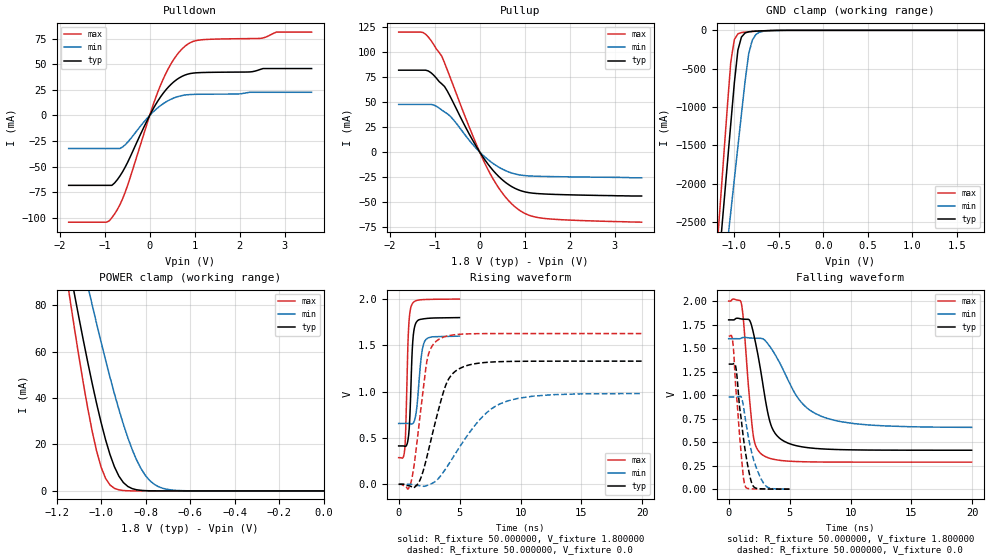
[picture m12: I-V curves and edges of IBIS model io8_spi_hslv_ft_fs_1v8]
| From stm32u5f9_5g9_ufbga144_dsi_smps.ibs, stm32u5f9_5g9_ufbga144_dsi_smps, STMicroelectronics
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|   Model io8_spi_hslv_ft_fs_1v8
[Model]  io8_spi_hslv_ft_fs_1v8
Model_type I/O
Polarity   Non-Inverting
Enable   Active-Low
Vinl =   0.540000V
Vinh =   1.260000V
Vmeas =  0.900000V
Cref =   50.000000pF
Rref =   100.000000M
Vref =   0.0V
C_comp   3.338700pF   3.332500pF   3.379000pF
[Temperature Range]   25.000000   0.140000k   -40.000000
[Pullup Reference]   1.800000V   1.600000V   2.000000V
[Pulldown Reference]   0.0V   0.0V   0.0V
[POWER Clamp Reference]   1.800000V   1.600000V   2.000000V
[GND Clamp Reference]   0.0V   0.0V   0.0V
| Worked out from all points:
|   slope of the pulldown table from 0 to 0.27 V, typ, clamps not added: 13.6 ohm
|   slope of the pullup table from 0 to 0.27 V, typ, clamps not added: 15.9 ohm
|   GND clamp passes 1 mA (typ) near -0.51 V on its own axis
|   POWER clamp passes 1 mA (typ) near -0.86 V on its own axis
|   rising waveform, R_fixture 50.000000, V_fixture 1.800000: 20-80 % time 245ps typ, 388ps min, 218ps max; typ from 0.414 V to 1.8 V
|   rising waveform, R_fixture 50.000000, V_fixture 0.0: 20-80 % time 1.59ns typ, 3.32ns min, 900ps max; typ from 0 V to 1.33 V
|   falling waveform, R_fixture 50.000000, V_fixture 1.800000: 20-80 % time 1.19ns typ, 2.71ns min, 660ps max; typ from 1.8 V to 0.414 V
|   falling waveform, R_fixture 50.000000, V_fixture 0.0: 20-80 % time 774ps typ, 1.04ns min, 578ps max; typ from 1.33 V to 0 V
[Pulldown]
|Voltage   I(typ)   I(min)   I(max)
-1.8V     -68.38mA   -32.32mA   -104.4mA
-960mV    -68.38mA   -32.32mA   -104.4mA
-780mV    -66.07mA   -32.32mA   -96.42mA
-540mV    -50.22mA   -28.51mA   -74.66mA
0V        0A         -300fA     0A
240mV     18.04mA    9.599mA    29.42mA
480mV     30.68mA    16.02mA    50.95mA
780mV     39.47mA    19.98mA    67.56mA
1.14V     41.99mA    20.78mA    74.01mA
2.46V     45.09mA    22.69mA    75.44mA
2.82V     45.91mA    22.69mA    81.6mA
3.6V      45.91mA    22.69mA    81.6mA
[Pullup]
|Voltage   I(typ)   I(min)   I(max)
-1.8V     82.11mA    47.76mA    120.3mA
-1.26V    82.11mA    47.76mA    120mA
-1.08V    79.5mA     47.76mA    111.8mA
-840mV    68.28mA    42.01mA    95.94mA
-660mV    56.17mA    36.23mA    75.42mA
-240mV    18.69mA    12.2mA     26.01mA
120mV     -8.174mA   -5.123mA   -11.83mA
480mV     -26.98mA   -16.65mA   -39.76mA
840mV     -37.65mA   -22.63mA   -57.07mA
1.08V     -40.74mA   -24.01mA   -63.22mA
1.44V     -42.19mA   -24.58mA   -66.73mA
3.6V      -44.2mA    -26mA      -70.5mA
[GND_clamp]
|Voltage   I(typ)   I(min)   I(max)
-1.8V     -9.908A    -9.683A    -9.994A
-1.2V     -3.383A    -4.084A    -2.934A
-1.16V    -2.841A    -3.655A    -2.294A
-1.12V    -2.299A    -3.226A    -1.656A
-1.04V    -1.218A    -2.369A    -414.2mA
-1V       -684.7mA   -1.941A    -119.2mA
-960mV    -257.2mA   -1.514A    -45.66mA
-920mV    -87.03mA   -1.089A    -28.93mA
-840mV    -19.35mA   -312.8mA   -18.96mA
-800mV    -13.55mA   -132.4mA   -15.49mA
-720mV    -8.042mA   -25.66mA   -9.49mA
1.8V      0A         13.64nA    0A
[POWER_clamp]
|Voltage   I(typ)   I(min)   I(max)
-1.8V     470.8mA    433.7mA    554.6mA
-1.14V    95.25mA    122.7mA    82.82mA
-1.12V    84.97mA    114mA      70.27mA
-1.06V    55.51mA    88.42mA    35.67mA
-1.04V    46.34mA    80.15mA    25.76mA
-1V       29.51mA    64.13mA    10.3mA
-940mV    10.39mA    41.86mA    1.109mA
-900mV    3.624mA    28.77mA    182.8uA
-840mV    490.7uA    13.24mA    11.35uA
-800mV    116.8uA    6.532mA    1.77uA
-740mV    13.2uA     1.724mA    109.3nA
0V        0A         18.75nA    0A
[Ramp]
| variable   typ   min   max
dV/dt_r  0.79770/1.58365n   0.58778/3.31184n   0.97662/0.89815n
dV/dt_f  0.83161/1.18880n   0.56477/2.70512n   1.02769/0.65829n
R_load = 50.000000
[Rising Waveform]
R_fixture= 50.000000
V_fixture= 1.800000
V_fixture_min= 1.600000
V_fixture_max= 2.000000
|time   V(typ)   V(min)   V(max)
0s        414mV      656.9mV    287.2mV
500.5ps   409.9mV    657mV      382.4mV
570.6ps   409.7mV    657.1mV    561.2mV
800.8ps   513.9mV    656.7mV    1.649V
920.9ps   742.1mV    654.9mV    1.855V
1.051ns   1.242V     651.6mV    1.931V
1.161ns   1.549V     655.7mV    1.958V
1.311ns   1.702V     695.4mV    1.975V
2.112ns   1.788V     1.538V     1.995V
4.985ns   1.8V       1.6V       2V
[Rising Waveform]
R_fixture= 50.000000
V_fixture= 0.0
V_fixture_min= 0.0
V_fixture_max= 0.0
|time   V(typ)   V(min)   V(max)
0s        -10.73uV   93.54nV    3.207uV
1.001ns   -22.8mV    -585.2uV   16.57mV
1.642ns   17.71mV    -14.22mV   611.5mV
2.322ns   299mV      -13.12mV   1.334V
3.283ns   812.3mV    65.66mV    1.564V
3.964ns   1.102V     187.9mV    1.601V
4.645ns   1.22V      328.7mV    1.616V
6.607ns   1.308V     690.7mV    1.627V
8.328ns   1.324V     868.7mV    1.628V
19.94ns   1.33V      980.3mV    1.628V
[Falling Waveform]
R_fixture= 50.000000
V_fixture= 1.800000
V_fixture_min= 1.600000
V_fixture_max= 2.000000
|time   V(typ)   V(min)   V(max)
0s        1.8V       1.6V       2V
1.041ns   1.809V     1.606V     1.974V
1.682ns   1.8V       1.608V     1.004V
2.002ns   1.676V     1.606V     586.4mV
2.803ns   1.119V     1.599V     361.9mV
3.363ns   727.6mV    1.52V      328.5mV
4.004ns   563mV      1.387V     310.1mV
5.766ns   456.2mV    954.6mV    292.9mV
7.608ns   428.6mV    774.6mV    288.6mV
19.94ns   414mV      656.9mV    287.2mV
[Falling Waveform]
R_fixture= 50.000000
V_fixture= 0.0
V_fixture_min= 0.0
V_fixture_max= 0.0
|time   V(typ)   V(min)   V(max)
0s        1.33V      980.3mV    1.628V
320.3ps   1.33V      980.4mV    1.581V
430.4ps   1.336V     980.5mV    1.424V
580.6ps   1.3V       980.4mV    1.081V
1.041ns   730.6mV    976.8mV    354mV
1.221ns   532.5mV    872.3mV    116.2mV
1.341ns   422.3mV    770.3mV    37.68mV
1.922ns   55.71mV    371.2mV    3.028mV
2.823ns   2.908mV    72.08mV    1.074mV
4.985ns   -10.73uV   93.54nV    3.207uV
